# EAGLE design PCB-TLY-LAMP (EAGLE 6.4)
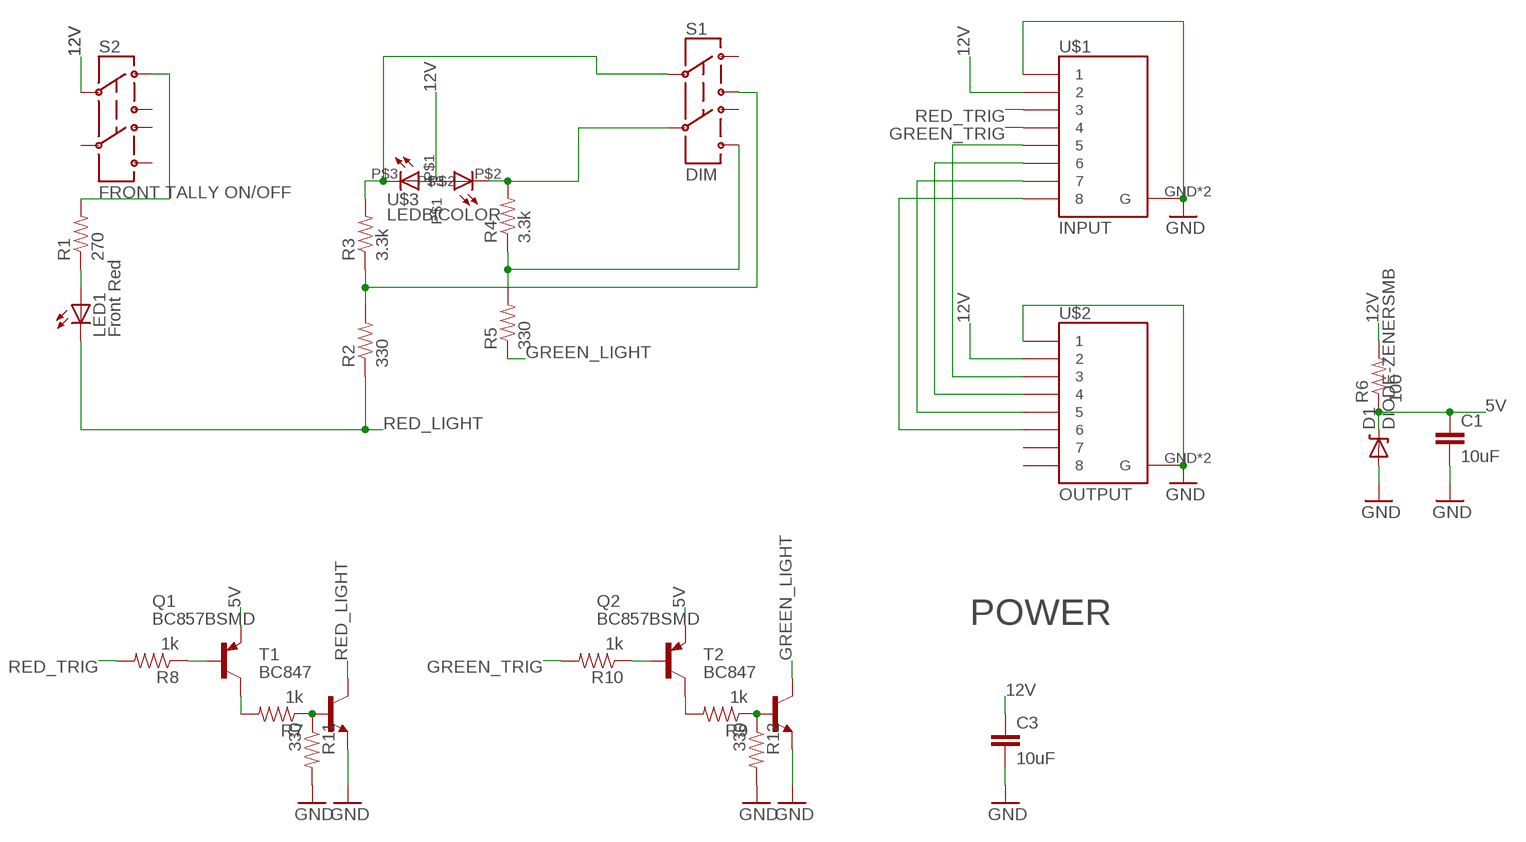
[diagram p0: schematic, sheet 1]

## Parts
C1  10uF  CAP0805  [0805]
C3  10uF  CAP0805  [0805]
D1  DIODE-ZENERSMB  [SMB-DIODE]
LED1  Front Red  LED20  [LED20]
Q1  BC857BSMD  [SOT23-BEC]
Q2  BC857BSMD  [SOT23-BEC]
R1  270  RESISTOR0603-RES  [0603-RES]
R2  330  RESISTOR0603-RES  [0603-RES]
R3  3.3k  RESISTOR0603-RES  [0603-RES]
R4  3.3k  RESISTOR0603-RES  [0603-RES]
R5  330  RESISTOR0603-RES  [0603-RES]
R6  100  RESISTOR0603-RES  [0603-RES]
R7  1k  RESISTOR0603-RES  [0603-RES]
R8  1k  RESISTOR0603-RES  [0603-RES]
R9  1k  RESISTOR0603-RES  [0603-RES]
R10  1k  RESISTOR0603-RES  [0603-RES]
R11  330  RESISTOR0603-RES  [0603-RES]
R12  330  RESISTOR0603-RES  [0603-RES]
S1  DIM  SWITCH-DPDTPTH1  [TECONNECTIVITY-DPDT]
S2  FRONT TALLY ON/OFF  SWITCH-DPDTPTH1  [TECONNECTIVITY-DPDT]
T1  BC847  [SOT23]
T2  BC847  [SOT23]
U$1  INPUT  RJ45-8_GND  [RJ45-8_GND]
U$2  OUTPUT  RJ45-8_GND  [RJ45-8_GND]
U$3  LEDBICOLOR  [LEDBICOLOR]

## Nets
5V: C1.1 D1.C Q1.E Q2.E R6.1
12V [POWER]: C3.1 R6.2 S2.P$2 U$1.2 U$2.2 U$3.P$1
GND [POWER]: C1.2 C3.2 D1.A R11.2 R12.2 T1.2(E) T2.2(E) U$1.1 U$1.GND1(G) U$1.GND(G) U$2.1 U$2.GND1(G) U$2.GND(G)
GREEN_LIGHT [POWER]: R5.1 T2.3(C)
GREEN_TRIG: R10.2 U$1.4
N$1 [POWER]: R1.2 S2.P$1
N$2 [POWER]: LED1.P$1(A) R1.1
N$3 [POWER]: R2.2 R3.1 S1.P$3
N$4 [POWER]: R4.1 R5.2 S1.P$6
N$5 [POWER]: R4.2 S1.P$5 U$3.P$2
N$6 [POWER]: R3.2 S1.P$2 U$3.P$3
N$7: U$1.5 U$2.3
N$8: U$1.6 U$2.4
N$9: R7.1 R11.1 T1.1(B)
N$10: Q1.C R7.2
N$11: U$1.7 U$2.5
N$12: U$1.8 U$2.6
N$13: R9.1 R12.1 T2.1(B)
N$14: Q2.C R9.2
N$15: Q2.B R10.1
N$16: Q1.B R8.1
RED_LIGHT [POWER]: LED1.P$2(C) R2.1 T1.3(C)
RED_TRIG: R8.2 U$1.3
Unconnected: S1.P$1 S1.P$4 S2.P$3 S2.P$4 S2.P$5 S2.P$6 U$2.7 U$2.8

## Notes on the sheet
- POWER

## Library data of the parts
C1 C3 = SparkFun:CAP: Capacitor
D1 = SparkFun:DIODE-ZENER: Zener Diode
LED1 = SKAARHOJ:LED20: KINGBRIGHT 20MM BIG LAMP
Q1 Q2 = transistor-pnp:BC857*: PNP Transistror
R1-R12 = SparkFun:RESISTOR: Resistor
S1 S2 = SKAARHOJ:SWITCH-DPDT: DPDT Version of the COM-00597
T1 T2 = transistor:BC847: NPN TRANSISTOR
U$1 U$2 = SKAARHOJ:RJ45-8_GND
U$3 = SKAARHOJ:LEDBICOLOR: L.C.LED N810TGLR2D 10mm Diffused Bicolor Led Lamp (Anode)

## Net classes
0 default: width 0.254 mm, drill 0.559 mm, clearance 0.203 mm
1 POWER: width 0.508 mm, drill 0.686 mm, clearance 0.203 mm

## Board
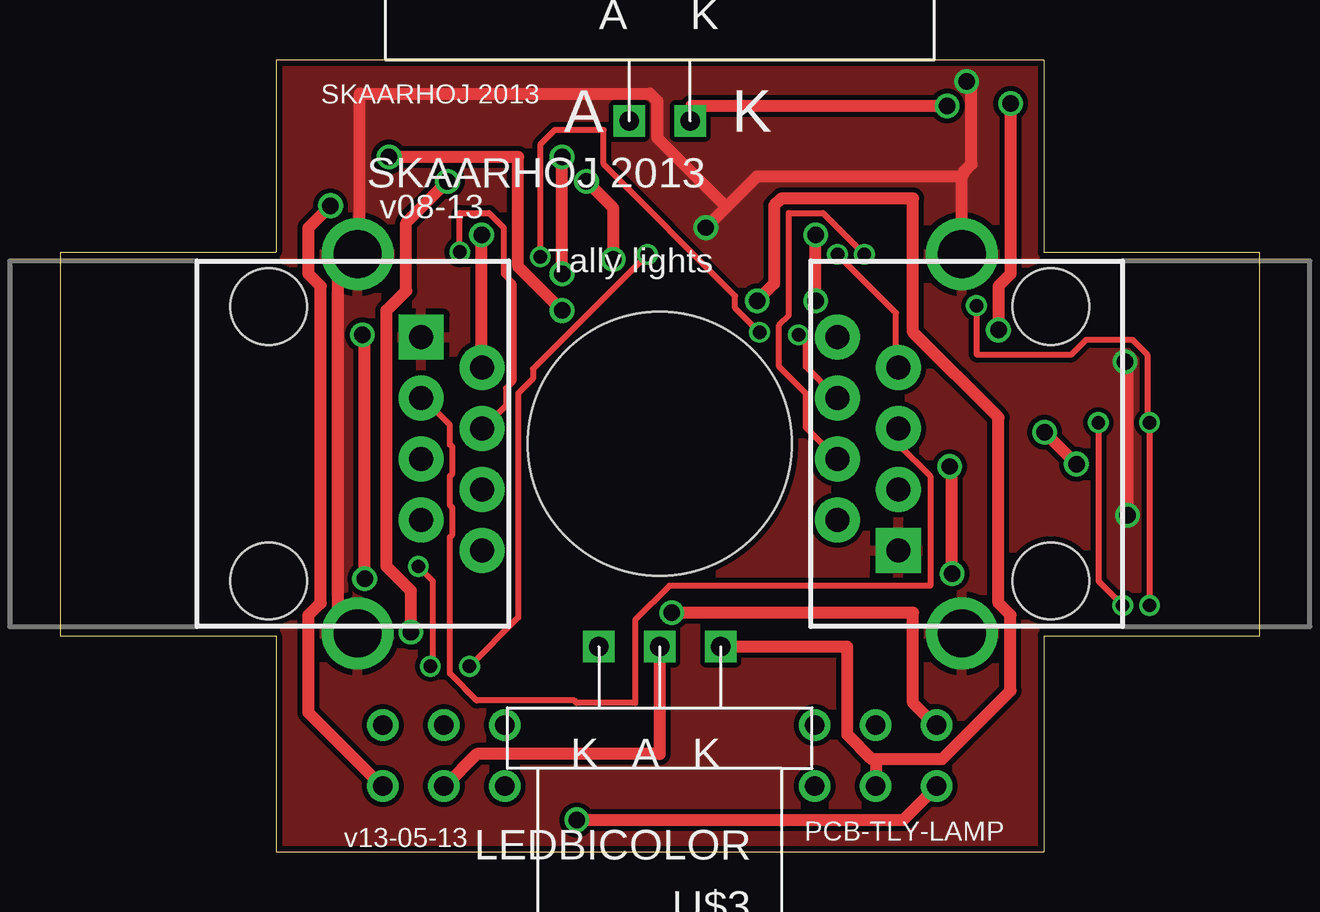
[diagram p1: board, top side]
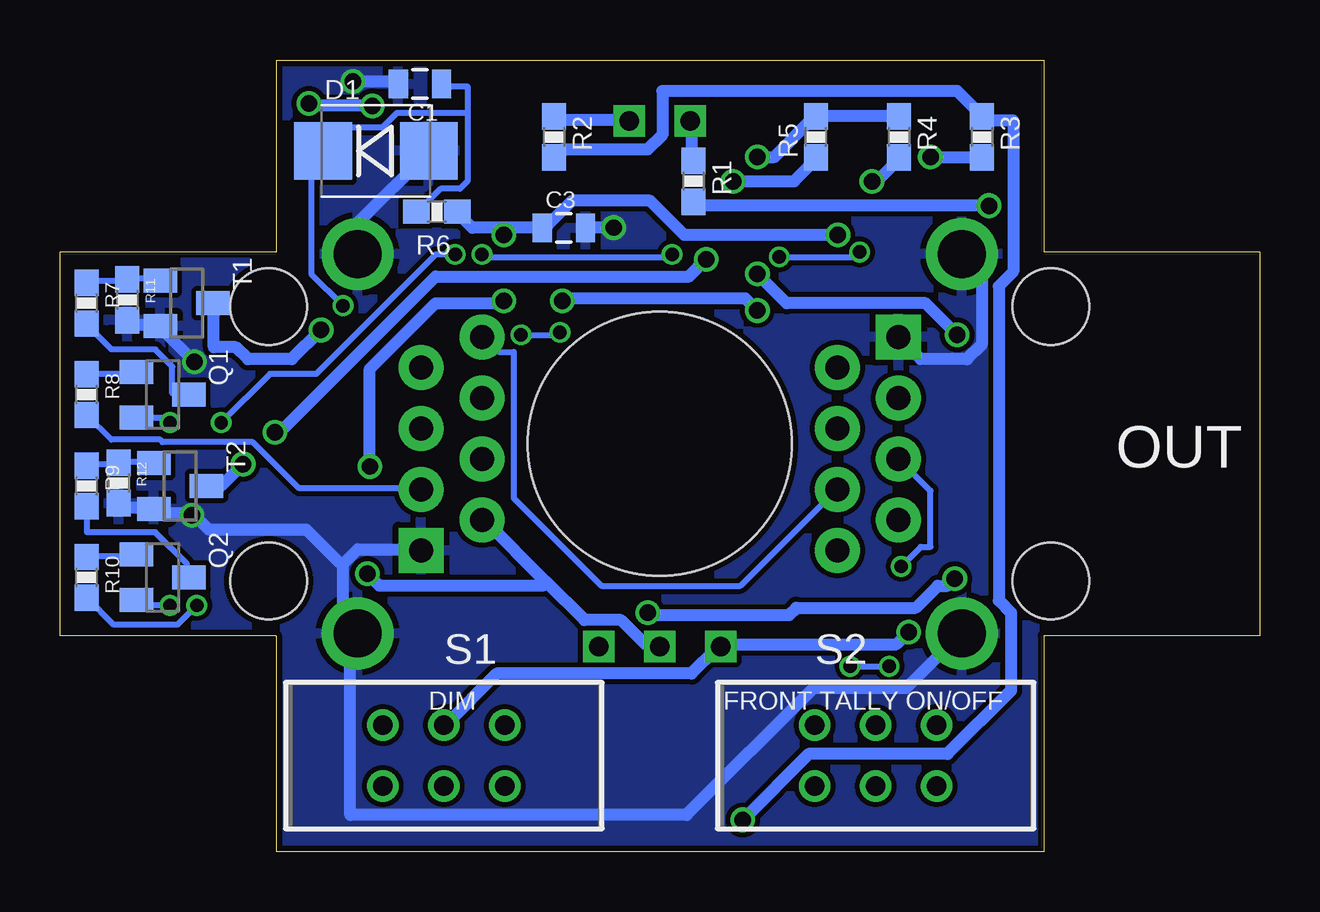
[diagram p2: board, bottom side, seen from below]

Size 50 x 33 mm. Coordinates in mm from the lower left corner, seen from the top.
Outline: 9,0 41,0 41,9 50,9 50,25 41,25 41,33 9,33 9,25 0,25 0,9 9,9 9,0
Copper layers (1*16): Top 0.035mm / dielectric 1.5mm / Bottom 0.035mm
Design rules "Fusion_eagle_rule_v1.1": minimum track width 6mil, minimum drill 12mil, track to track 6mil, track to pad 6mil, pad to pad 6mil, via to via 6mil, smd to smd 0mil, copper to edge 10mil, drill to drill 10mil, minimum pad ring 10mil, minimum via ring 6mil, stop-mask expansion 2mil, vias tented up to drill 100mil, thermal gap 10mil
Holes 11 mm at 25,17

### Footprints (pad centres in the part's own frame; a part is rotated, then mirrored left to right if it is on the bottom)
0805 = smd 0.8 x 1.2: 1 -0.9,0; 2 0.9,0
SMB-DIODE = smd 2.4 x 2.4: A 2.2,0; C -2.2,0
LED20 = drill 0.8 square: P$1 -1.27,-2.54; P$2 1.27,-2.54
SOT23-BEC = smd 1 x 1.4: B -0.95,-1.1; C 0,1.1; E 0.95,-1.1
0603-RES = smd 1.1 x 1: 1 -0.85,0; 2 0.85,0
TECONNECTIVITY-DPDT = drill 0.8: P$1 1.27,2.54; P$2 1.27,0; P$3 1.27,-2.54; P$4 -1.27,2.54; P$5 -1.27,0; P$6 -1.27,-2.54
SOT23 = smd 1 x 1.4: 1 -0.95,-1.1; 2 0.95,-1.1; 3 0,1.1
RJ45-8_GND = drill 1 pad 1.88 square: 1 -4.445,6.35 | drill 1 pad 1.88: 2 -3.175,8.89; 3 -1.905,6.35; 4 -0.635,8.89; 5 0.635,6.35; 6 1.905,8.89; 7 3.175,6.35; 8 4.445,8.89 | drill 2: GND -7.9,3.7; GND1 7.9,3.7 | hole 3.2: -5.715,0; 5.715,0
LEDBICOLOR = drill 0.8 square: P$1 0,-2.54; P$2 2.54,-2.54; P$3 -2.54,-2.54

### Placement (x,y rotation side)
C1  35,32 180 bottom
C3  29,26 0 bottom
D1  36.83,29.21 0 bottom
LED1  25,33 0 top
Q1  45.72,19.05 270 bottom
Q2  45.72,11.43 270 bottom
R1  23.59,27.94 270 bottom
R2  29.41,29.79 270 bottom
R3  11.57,29.79 270 bottom
R4  15.03,29.79 270 bottom
R5  18.49,29.79 90 bottom
R6  34.29,26.67 0 bottom
R7  48.9,22.86 270 bottom
R8  48.9,19.05 270 bottom
R9  48.9,15.24 270 bottom
R10  48.9,11.43 270 bottom
R11  47.19,23 270 bottom
R12  47.55,15.37 270 bottom
S1  34,4 270 bottom
S2  16,4 270 bottom
T1  44.72,22.86 270 bottom
T2  44.99,15.24 270 bottom
U$1  41.3,17 90 top
U$2  8.7,17 270 top
U$3  25,6 180 top

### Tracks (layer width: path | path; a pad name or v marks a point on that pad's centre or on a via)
5V  (via drill 0.56)
  Top 0.254: v45.41,10.26 v45.41,17.88 45.41,17.98 45.31,18.09 45.31,20.73 44.7,21.34 42.77,21.34 42.16,20.73 38.2,20.73 v38.2,22.76
  Bottom 0.254: v45.41,10.26 46.53,10.26 46.74,10.46 Q2.E | v45.41,17.88 45.62,18.09 46.74,18.09 Q1.E | 33.02,30.79 33.02,31.9 34.04,31.9 C1.1 | 33.02,30.79 33.02,27.94 33.33,27.64 34.14,27.64 35.05,26.72 R6.1 | 33.02,30.79 35.97,30.79 36.58,30.18 38.1,30.18 39.01,29.26 D1.C 39.12,29.16 39.52,29.16 39.52,24.08 v38.2,22.76
12V  (via drill 0.69)
  Top 0.508: v17.58,25.7 17.58,20.22 U$2.2 | S2.P$2 16.05,2.74 17.37,4.06 24.99,4.06 U$3.P$1 | v31.5,22.96 v31.5,25.7 | v37.08,16.05 37.19,15.95 v37.19,11.58
  Bottom 0.508: 31.5,26.01 29.97,26.01 C3.1 29.67,26.11 28.65,27.13 25.4,27.13 23.98,25.7 v17.58,25.7 | 31.5,26.01 32.82,26.01 33.43,26.62 R6.2 | 29.72,11.23 28.14,9.65 26.62,9.65 25.6,8.64 25.09,8.64 U$3.P$1 | 29.72,11.23 32.31,13.82 U$1.2 | v31.5,22.96 31.6,22.86 34.34,22.86 37.08,20.12 v37.08,16.05 | v37.19,11.58 36.68,11.07 29.87,11.07 29.72,11.23 | v31.5,25.7 31.5,26.01
GND  (via drill 0.69)
  Top 0.508: v44.4,20.42 44.5,20.32 v44.5,14.02 | 27.79,26.87 29.06,28.14 37.59,28.14 | 27.79,26.87 v26.92,26.01 | 37.59,28.14 37.59,24.99 U$1.GND1 | v37.8,32.11 38,31.9 38,28.65 37.69,28.35 37.59,28.14 | U$2.GND1 12.39,9.14 11.58,9.96 11.58,24.08 U$2.GND 12.5,25.09 12.5,31.6 24.59,31.6 24.89,31.29 24.89,29.77 27.79,26.87
  Bottom 0.508: R11.2 47.14,22.15 46.94,21.95 45.82,21.95 T1.2 45.72,21.74 v44.4,20.42 | R12.2 47.55,14.43 47.45,14.33 46.13,14.33 T2.2 45.92,14.12 44.6,14.12 v44.5,14.02 44.3,13.92 43.79,13.41 39.73,13.41 38.41,12.09 38.2,11.99 | 38.2,11.99 37.59,12.6 34.95,12.6 U$1.1 | 38.2,11.99 38.2,9.14 37.69,9.14 U$1.GND 37.9,8.94 37.9,1.52 23.88,1.52 18.59,6.81 14.73,6.81 12.5,9.04 U$2.GND1 | v26.92,26.01 28.04,26.01 C3.2 | v37.8,32.11 36.07,32.11 35.97,32 C1.2 | D1.A 34.65,29.16 37.59,26.21 37.59,24.99 U$1.GND1 | U$2.1 15.04,21.44 14.12,20.52 12.19,20.52 11.58,21.13 11.58,24.89 U$2.GND
  pour Top: 0,0 50,0 50,33 0,33
  pour Bottom: 0,0 50,0 50,33 0,33
GREEN_LIGHT  (via drill 0.69)
  Top 0.508: v21.95,27.94 23.06,26.82 v23.06,24.69 | v42.37,16.15 v41.05,17.48
  Bottom 0.508: v21.95,27.94 19.41,27.94 18.49,28.85 R5.1 | v23.06,24.69 23.77,23.98 34.34,23.98 40.84,17.48 v41.05,17.48 | v42.37,16.15 43.28,15.24 T2.3
GREEN_TRIG  (via drill 0.56)
  Top 0.254: v44.3,10.26 43.28,11.28 v43.28,17.88 | v33.53,24.89 31.8,26.62 30.38,26.62 30.38,22.35 29.97,21.95 29.97,20.22 31.09,19.1 31.09,17.68 32.31,16.46 U$1.4
  Bottom 0.254: v44.3,10.26 45.11,9.45 47.75,9.45 48.87,10.57 R10.2 | v43.28,17.88 41.25,19.91 39.32,19.91 34.34,24.89 v33.53,24.89
N$1  (via drill 0.69)
  Top 0.508: v11.28,26.92 10.36,26.01 10.36,24.08 10.87,23.57 10.87,10.36 10.36,9.86 10.36,5.79 13.41,2.74 S2.P$1
  Bottom 0.508: v11.28,26.92 23.47,26.92 23.57,27.03 R1.2
N$2
  Bottom 0.508: R1.1 23.67,28.85 23.67,30.38 LED1.P$1
N$3  (via drill 0.69)
  Top 0.508: v21.54,1.32 35.15,1.32 36.47,2.64 S1.P$3
  Bottom 0.508: R2.2 29.36,28.96 29.06,29.26 25.5,29.26 24.89,29.87 24.89,31.7 12.6,31.7 11.58,30.68 R3.1 11.38,30.48 10.26,30.48 10.26,24.18 10.87,23.57 10.87,10.46 10.36,9.96 10.36,6.71 13.01,4.06 18.8,4.06 v21.54,1.32
N$4  (via drill 0.69)
  Top 0.508: v20.93,24.08 v20.93,28.96 | v12.6,21.54 12.7,21.44 v12.7,11.38 | v25.5,9.96 35.56,9.96 35.56,6.2 36.47,5.28 S1.P$6
  Bottom 0.508: R4.1 15.04,30.68 18.39,30.68 R5.2 18.69,30.48 20.22,28.96 v20.93,28.96 | v20.93,24.08 19.71,22.86 13.92,22.86 v12.6,21.54 | v12.7,11.38 13.01,11.07 13.41,11.07 14.33,10.16 19.3,10.16 19.61,9.86 25.4,9.86 v25.5,9.96
N$5  (via drill 0.69)
  Top 0.508: v16.15,27.94 14.43,26.21 14.43,23.37 13.61,22.55 13.61,11.89 14.63,10.87 v14.63,9.14
  Bottom 0.508: v16.15,27.94 15.95,27.94 15.04,28.85 R4.2 | v14.63,9.14 15.14,8.64 22.45,8.64 U$3.P$2 22.66,8.43 23.67,7.42 31.8,7.42 33.93,5.28 S1.P$5
N$6  (via drill 0.69)
  Top 0.508: v13.72,28.96 19.1,28.96 19.1,24.38 v20.93,22.55 | v29.06,22.96 29.77,23.67 29.77,26.92 30.07,27.23 35.56,27.23 35.56,21.64 39.12,18.09 39.12,10.36 39.62,9.86 39.62,6.71 36.78,3.86 34.04,3.86 | 34.04,3.86 34.04,2.74 S1.P$2 | U$3.P$3 27.64,8.53 32.82,8.53 32.82,4.88 33.83,3.86 34.04,3.86
  Bottom 0.508: v13.72,28.96 11.58,28.96 R3.2 | v20.93,22.55 21.44,23.06 28.96,23.06 v29.06,22.96
N$7
  Top 0.254: U$2.3 15.14,18.9 16.26,17.78 16.26,16.97 16.36,16.87 16.36,15.75 16.26,15.65 16.26,14.43 16.36,14.33 16.36,13.21 16.26,13.11 16.26,7.42 17.37,6.3 21.44,6.3 21.54,6.2 23.98,6.2 23.98,9.65 25.4,11.07 36.27,11.07 36.27,15.65 34.95,16.97 34.95,17.58 U$1.5
N$8  (via drill 0.56)
  Top 0.254: v16.66,24.99 16.66,26.62 17.88,26.62 18.49,26.01 18.49,24.08 18.9,23.67 18.9,19.61 18.59,19.3 18.59,18.59 17.68,17.68 U$2.4 | v20.02,24.79 20.02,29.46 20.62,30.07 22.66,30.07 22.66,28.65 28.14,23.16 28.14,22.66 v29.16,21.64 | v30.79,21.54 31.09,21.23 31.09,20.22 32.31,19 U$1.6
  Bottom 0.254: v16.66,24.99 16.87,24.79 v20.02,24.79 | v29.16,21.64 29.26,21.54 v30.79,21.54
N$9
  Bottom 0.254: T1.1 45.82,23.88 47.14,23.88 R11.1 47.24,23.77 48.87,23.77 R7.1
N$10
  Bottom 0.254: R7.2 48.87,21.95 47.85,20.93 46.02,20.93 45.31,20.22 45.31,19.1 44.7,19.1 Q1.C
N$11  (via drill 0.56)
  Top 0.254: v14.94,11.89 15.54,11.28 15.54,7.82 v15.44,7.72 | v17.07,7.72 19.1,9.75 19.1,19.1 19.71,19.71 19.71,20.12 v24.49,24.89 | v32.41,24.89 34.85,22.45 34.85,20.22 U$1.7
  Bottom 0.254: v14.94,11.89 14.12,12.7 13.72,12.7 13.72,15.04 15.04,16.36 U$2.5 | v17.07,7.72 v15.44,7.72 | v24.49,24.89 24.59,24.79 32.31,24.79 v32.41,24.89
N$12
  Bottom 0.254: U$2.6 17.68,15.04 21.64,11.07 27.43,11.07 31.09,14.73 31.09,20.83 31.7,20.83 32.31,21.44 U$1.8
N$13
  Bottom 0.254: R9.1 48.87,16.15 47.65,16.15 R12.1 47.45,16.26 46.13,16.26 T2.1
N$14
  Bottom 0.254: R9.2 48.87,14.33 48.87,13.31 46.02,13.31 44.7,11.99 44.7,11.48 Q2.C
N$15
  Bottom 0.254: R10.1 48.87,12.29 46.84,12.29 Q2.B
N$16
  Bottom 0.254: R8.1 48.87,19.91 46.84,19.91 Q1.B
RED_LIGHT  (via drill 0.69)
  Top 0.508: v39.12,21.74 39.12,23.57 39.62,24.08 v39.62,31.19 | v36.98,31.09 26.31,31.09 26.31,30.48 LED1.P$2
  Bottom 0.508: R2.1 29.36,30.58 29.26,30.48 26.31,30.48 LED1.P$2 | v39.12,21.74 40.34,20.52 42.16,20.52 42.67,21.03 43.59,21.03 43.59,22.86 T1.3 | v39.62,31.19 39.52,31.09 v36.98,31.09
RED_TRIG
  Bottom 0.254: R8.2 48.87,18.19 47.85,17.17 45.82,17.17 45.72,17.07 41.96,17.07 40.03,15.14 34.95,15.14 U$1.3

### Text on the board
_tsilk: SKAARHOJ 2013 | A | K | SKAARHOJ 2013 | v08-13 | Tally lights | v13-05-13 | PCB-TLY-LAMP
_bsilk: OUT

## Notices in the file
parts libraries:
SparkFun: Licensing: CC v3.0 Share-Alike You are welcome to use this library for commercial purposes.
